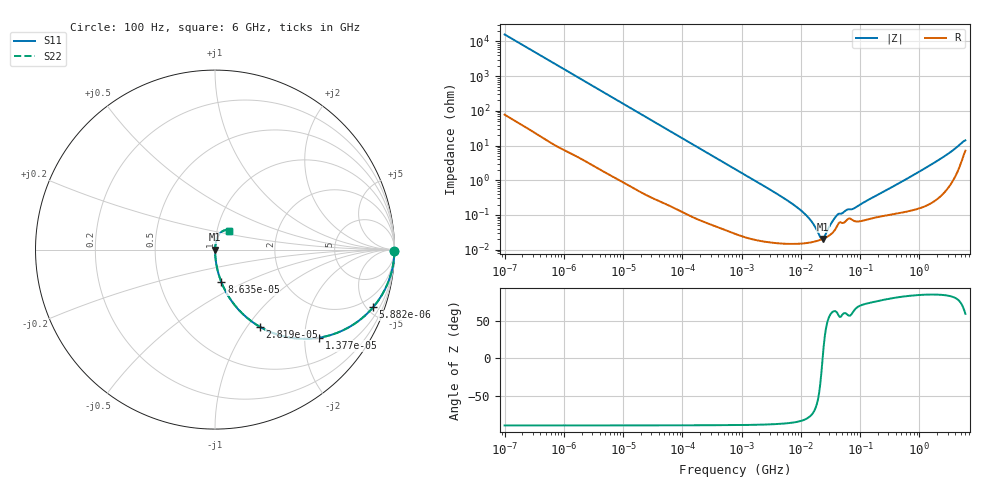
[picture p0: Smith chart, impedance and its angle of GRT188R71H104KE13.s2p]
!Murata Part Number: GRT188R71H104KE13
!These Parameters are Measured in Series Mode Connection
!Data Generated on Jun 19, 2026
!  o--ll--o
!Port1  Port2
!  o------o
!Operation Temp=25[degC], DC Bias Voltage=0[V]
!Freq. Start=100[Hz] Stop=6[GHz] 401[Steps]
# Hz S RI R 50
!Freq.(Hz) S11(Real) S11(Imag) S21(Real) S21(Imag) S12(Real) S12(Imag) S22(Real) S22(Imag)
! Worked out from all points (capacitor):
!   401 points, 100 Hz to 6 GHz, reference 50 ohm
!   read as one part in series: C = 99.8 nF near 109 Hz
!   lowest |Z| = 20.3 mohm at 23.28 MHz (marker M1)
!   series resonance near 23.32 MHz, so ESL is about 470 pH
!   S11 on the Smith chart (normalised r, x): 100 Hz: open; 5.882 kHz: 1.03, -5.48; 13.77 kHz: 1.01, -2.35; 28.19 kHz: 1.01, -1.15; 86.35 kHz: 1.00, -0.38; 6 GHz: 1.14, +0.24
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100  0.9999 -0.00628  7e-05 0.00628  7e-05 0.00628  0.9999 -0.00628
627  0.9983 -0.0391  0.00171 0.0391  0.00171 0.0391  0.9983 -0.0391
2008  0.984 -0.1229  0.016 0.1229  0.016 0.1229  0.984 -0.1229
5882  0.8813 -0.3208  0.1187 0.3208  0.1187 0.3208  0.8813 -0.3208
13772  0.5793 -0.4909  0.4207 0.4909  0.4207 0.4909  0.5793 -0.4909
28191  0.2497 -0.43  0.7503 0.43  0.7503 0.43  0.2497 -0.43
40335  0.1409 -0.3448  0.8591 0.3448  0.8591 0.3448  0.1409 -0.3448
86348  0.0356 -0.1816  0.9644 0.1816  0.9644 0.1816  0.0356 -0.1816
221108  0.00607 -0.0734  0.9939 0.0734  0.9939 0.0734  0.00607 -0.0734
774597  0.000736 -0.0212  0.9993 0.0212  0.9993 0.0212  0.000736 -0.0212
6948629  0.000151 -0.00218  0.9998 0.00218  0.9998 0.00218  0.000151 -0.00218
1.137099e7  0.000153 -0.00111  0.9998 0.00111  0.9998 0.00111  0.000153 -0.00111
1.555665e7  0.000165 -0.000593  0.9998 0.000593  0.9998 0.000593  0.000165 -0.000593
2.128304e7  0.000191 -0.000131  0.9998 0.000131  0.9998 0.000131  0.000191 -0.000131
2.327686e7  0.000202 -2.5e-06  0.9998 2.5e-06  0.9998 2.5e-06  0.000202 -2.5e-06
2.545746e7  0.000217 0.000127  0.9998 -0.000127  0.9998 -0.000127  0.000217 0.000127
3.482834e7  0.000315 0.000609  0.9997 -0.000609  0.9997 -0.000609  0.000315 0.000609
4.165952e7  0.000508 0.00089  0.9995 -0.00089  0.9995 -0.00089  0.000508 0.00089
8.154455e7  0.000663 0.00145  0.9993 -0.00145  0.9993 -0.00145  0.000663 0.00145
3.124326e8  0.00104 0.00569  0.999 -0.00569  0.999 -0.00569  0.00104 0.00569
1.873145e9  0.00373 0.0334  0.9963 -0.0334  0.9963 -0.0334  0.00373 0.0334
6e9  0.0787 0.1052  0.9213 -0.1052  0.9213 -0.1052  0.0787 0.1052
